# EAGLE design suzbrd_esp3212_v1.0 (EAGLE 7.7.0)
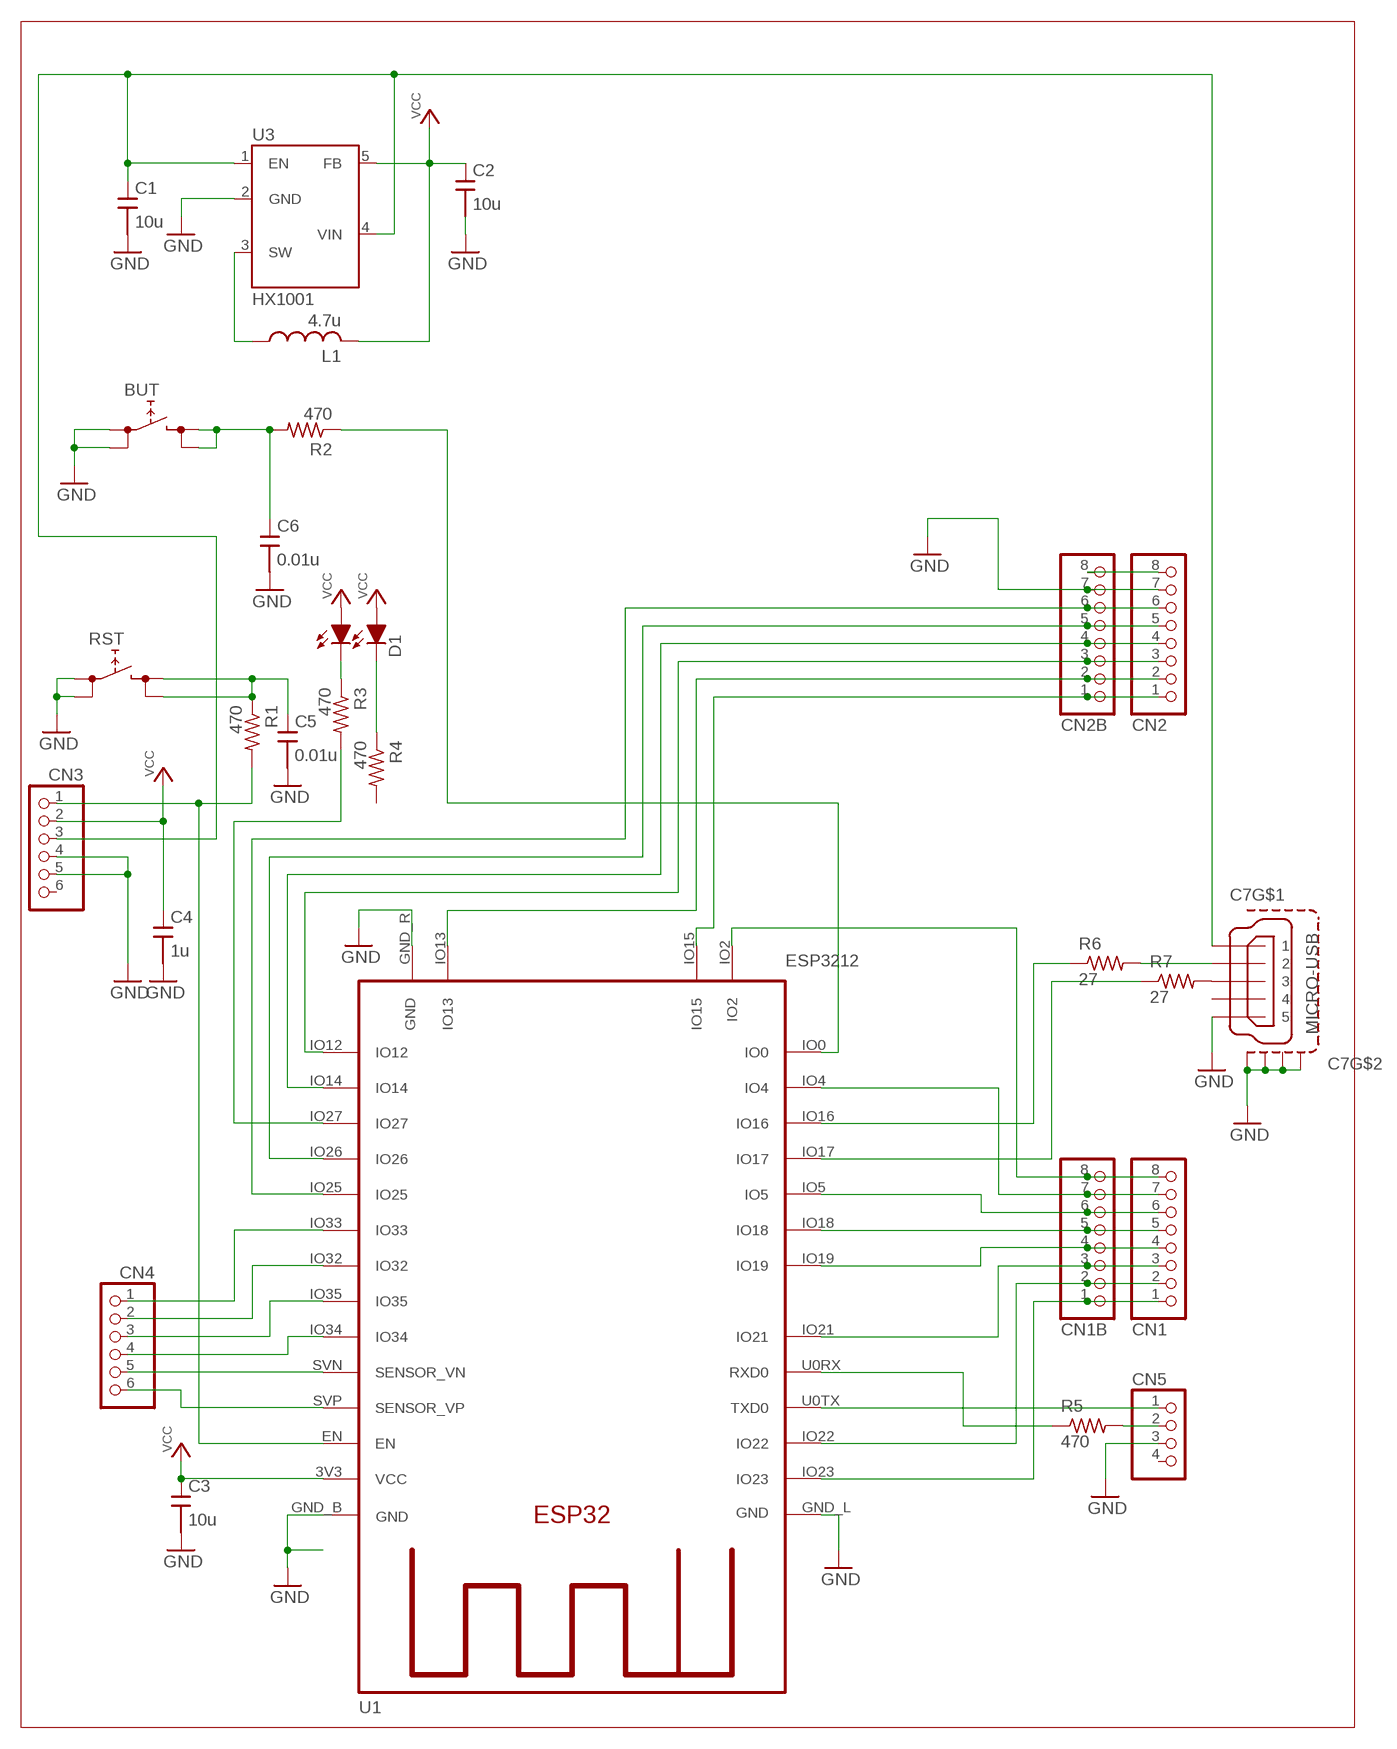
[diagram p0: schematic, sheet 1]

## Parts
BUT  TACTSWSMD+  [TACTSW/SMD+]
C1  10u  C/SMDC2012  [C2012]
C2  10u  C/SMDC2012  [C2012]
C3  10u  C/SMDC2012  [C2012]
C4  1u  C/SMDC2012  [C2012]
C5  0.01u  C/SMDC2012  [C2012]
C6  0.01u  C/SMDC2012  [C2012]
C7  MICRO-USB  [ZX62R]
CN1  PINHDR8  [PINHDR1X8]
CN1B  PINHDR81.0  [PINHDR1X8_1.0]
CN2  PINHDR8  [PINHDR1X8]
CN2B  PINHDR81.0  [PINHDR1X8_1.0]
CN3  PINHDR61.0  [PINHDR1X6_1.0]
CN4  PINHDR61.0  [PINHDR1X6_1.0]
CN5  CONN4N  [PINHDR1X4]
D1  SEC2XX4  [LED3025]
L1  4.7u  L/SMDNRG4026  [NRG4026]
R1  470  R/SMDR2012  [R2012]
R2  470  R/SMDR2012  [R2012]
R3  470  R/SMDR2012  [R2012]
R4  470  R/SMDR2012  [R2012]
R5  470  R/SMDR2012  [R2012]
R6  27  R/SMDR2012  [R2012]
R7  27  R/SMDR2012  [R2012]
RST  TACTSWSMD+  [TACTSW/SMD+]
U1  ESP3212  [ESP3212]
U3  HX1001  [SOT235]

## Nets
5V: C1.1 C7.1 CN3.3 U3.1(EN) U3.4(VIN)
EN: CN3.1 R1.2 U1.EN
GND: BUT.1 BUT.2 C1.2 C2.2 C3.2 C4.2 C5.2 C6.2 C7.5 C7.M1(S1) C7.M2(S2) C7.M3(S3) C7.M4(S4) CN2.7 CN2B.7 CN3.4 CN3.5 CN5.3 RST.1 RST.2 U1.GND_B(GND) U1.GND_L(GND) U1.GND_R(GND) U3.2(GND)
IO0: R2.1 U1.IO0
IO2: CN1.8 CN1B.8 U1.IO2
IO4: CN1.7 CN1B.7 U1.IO4
IO5: CN1.6 CN1B.6 U1.IO5
IO12: CN2.3 CN2B.3 U1.IO12
IO13: CN2.2 CN2B.2 U1.IO13
IO14: CN2.4 CN2B.4 U1.IO14
IO15: CN2.1 CN2B.1 U1.IO15
IO16: R6.1 U1.IO16
IO17: R7.1 U1.IO17
IO18: CN1.5 CN1B.5 U1.IO18
IO19: CN1.4 CN1B.4 U1.IO19
IO21: CN1.3 CN1B.3 U1.IO21
IO22: CN1.2 CN1B.2 U1.IO22
IO23: CN1.1 CN1B.1 U1.IO23
IO25: CN2.6 CN2B.6 U1.IO25
IO26: CN2.5 CN2B.5 U1.IO26
IO27: R3.2 U1.IO27
IO32: CN4.2 U1.IO32
IO33: CN4.1 U1.IO33
IO34: CN4.4 U1.IO34
IO35: CN4.3 U1.IO35
N$1: C7.3 R7.2
N$3: CN5.2 R5.2
N$21: C5.1 R1.1 RST.3 RST.4
N$25: D1.2(C1) R3.1
N$26: D1.1(C0) R4.1
N$32: C7.2 R6.2
N$36: CN2.8 CN2B.8
N$37: BUT.3 BUT.4 C6.1 R2.2
RXD0: R5.1 U1.U0RX(RXD0)
SW: L1.1 U3.3(SW)
TXD0: CN5.1 U1.U0TX(TXD0)
VCC: C2.1 C3.1 C4.1 CN3.2 D1.3(A1) D1.4(A0) L1.2 U1.3V3(VCC) U3.5(FB)
VN: CN4.5 U1.SVN(SENSOR_VN)
VP: CN4.6 U1.SVP(SENSOR_VP)
Unconnected: C7.4 CN3.6 CN5.4 R4.2

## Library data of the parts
BUT RST = SRT162-010:TACTSW: 4pin tactsw (1,2 - 3,4)
C1-C6 = SRT162-010:C/SMD
C7 = SRT162-020:MICRO-USB
CN1 CN1B CN2 CN2B = SRT162-010:PINHDR8
CN3 CN4 = SRT162-010:PINHDR6
CN5 = SRT162-010:CONN4: connector 4
D1 = SRT162-010:SEC2XX4
L1 = SRT162-010:L/SMD: VLF4012AT
R1-R7 = SRT162-010:R/SMD
U1 = SRT162-020:ESP3212
U3 = SRT162-010:HX1001

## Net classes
1 Power: width 0.381 mm, clearance 0.203 mm to class 0

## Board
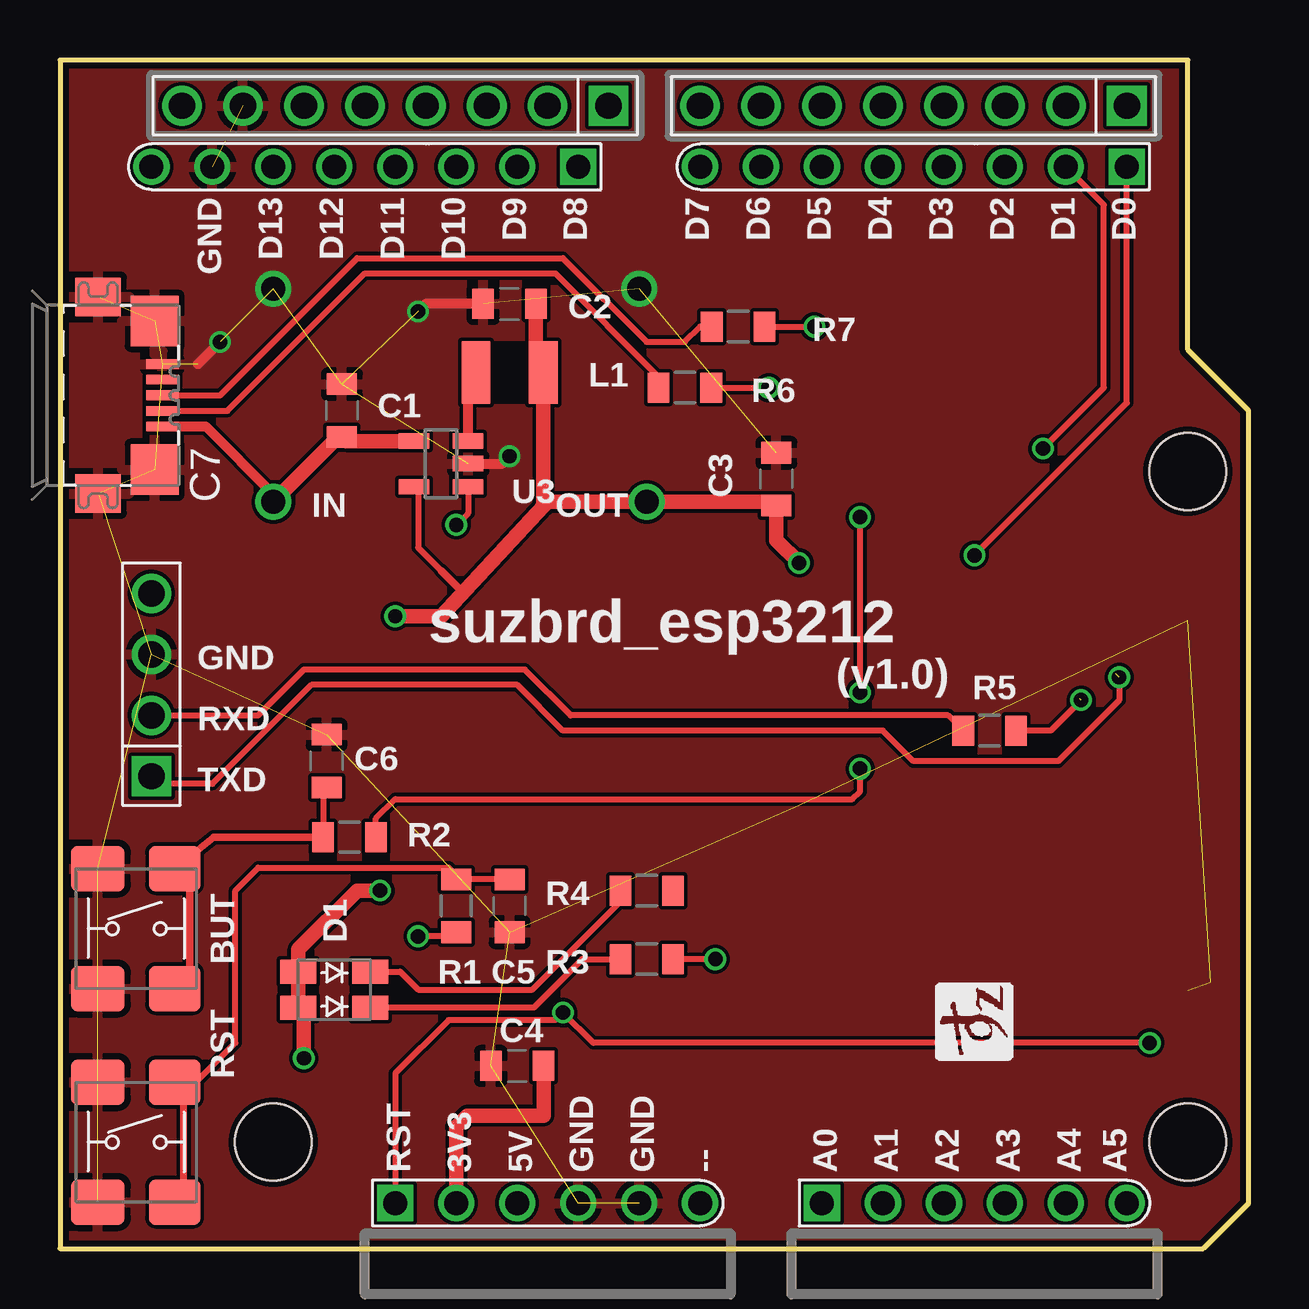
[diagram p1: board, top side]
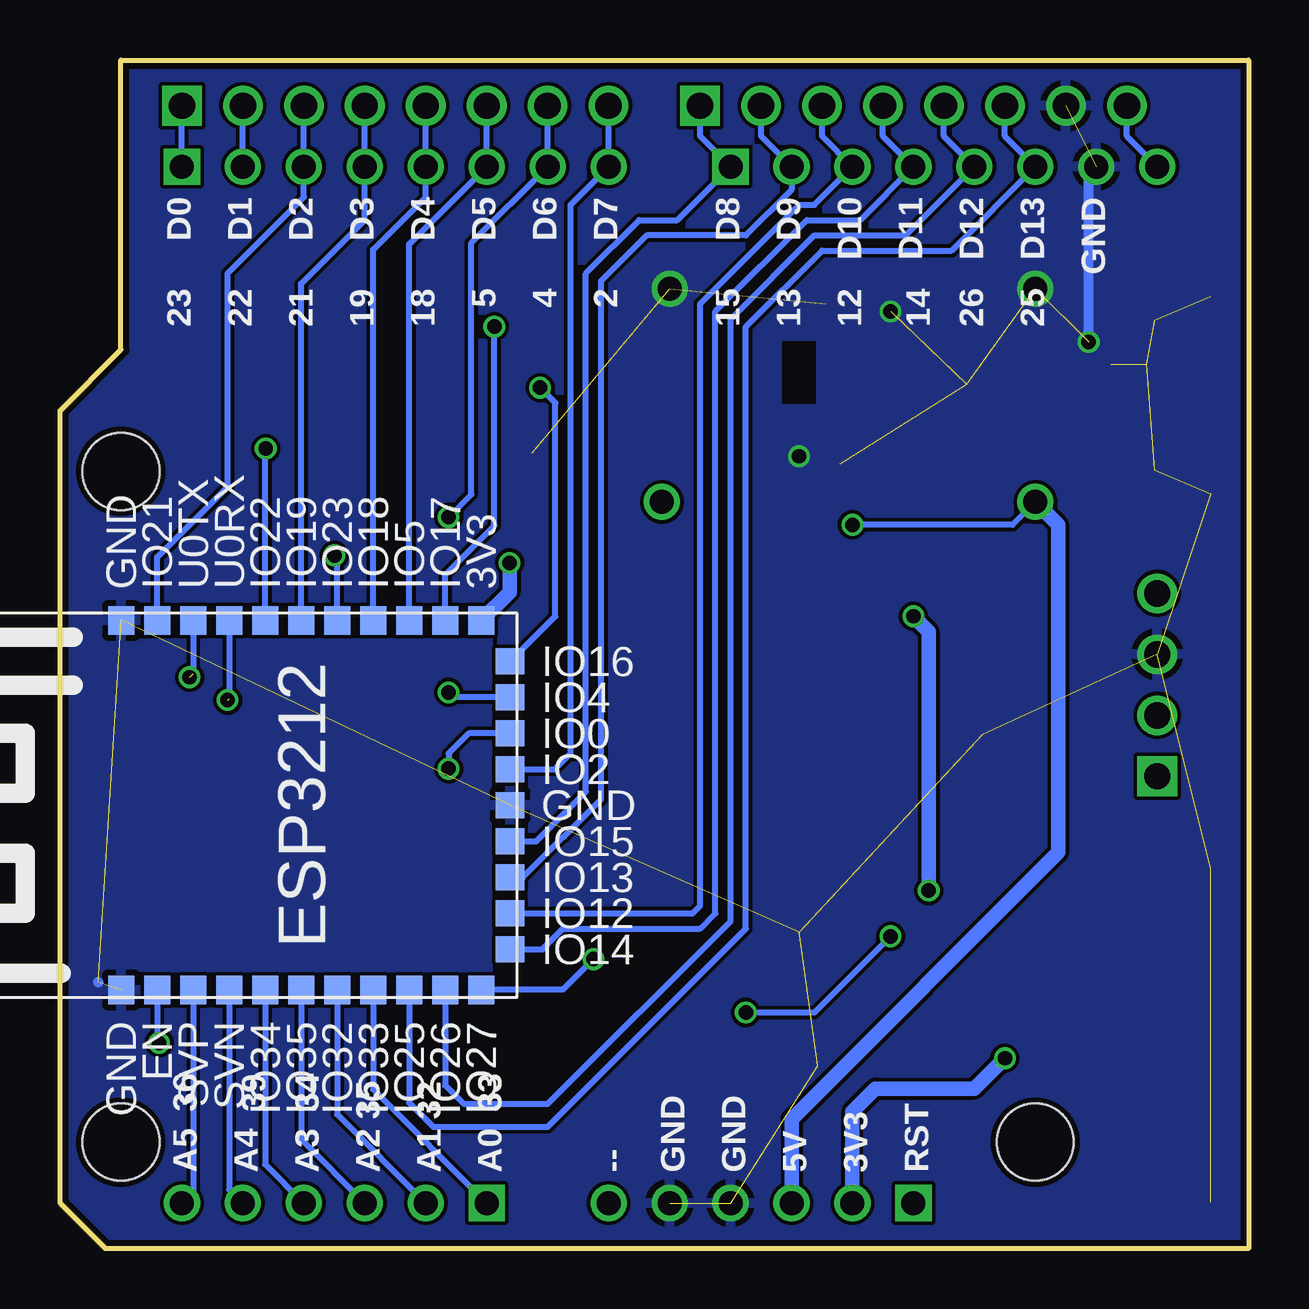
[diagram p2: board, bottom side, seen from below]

Size 49.53 x 49.53 mm. Coordinates in mm from the lower left corner, seen from the top.
Outline: 0,0 47.62,0 49.53,1.91 49.53,34.93 46.99,37.47 46.99,49.53 0,49.53 0,0
Copper layers (1*16): Top 0.035mm / dielectric 1.5mm / Bottom 0.035mm
Design rules "SeeedStudio": minimum track width 6mil, minimum drill 12mil, track to track 6mil, track to pad 6mil, pad to pad 6mil, via to via 6mil, smd to smd 0mil, copper to edge 10mil, drill to drill 10mil, minimum pad ring 10mil, minimum via ring 6mil, stop-mask expansion 2mil, vias tented up to drill 25mil, thermal gap 10mil
Holes 3.2 mm at 46.99,4.45 46.99,32.39 8.89,4.45
vRestrict: area 1.9,41.9 to 45.7,44.5; area 12.7,3.2 to 44.4,5.1

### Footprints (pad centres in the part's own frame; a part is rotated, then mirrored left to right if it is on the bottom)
TACTSW/SMD+ = smd 2.25 x 1.9: 1 -1.6,2.5; 2 -1.6,-2.5 | smd 2.15 x 1.9: 3 1.6,2.5; 4 1.6,-2.5
C2012 = smd 0.9 x 1.25: 1 -1.1,0; 2 1.1,0
ZX62R = smd 1.35 x 0.4: 1 2.675,-1.3; 2 2.675,-0.65; 3 2.675,0; 4 2.675,0.65; 5 2.675,1.3 | smd 1.9 x 1.6: M1 0,-4.1; M2 0,4.1 | smd 2 x 2.1: M3 2.35,3.1; M4 2.35,-3.1
PINHDR1X8 = drill 1.1 square: 1 -8.89,0 | drill 1.1: 2 -6.35,0; 3 -3.81,0; 4 -1.27,0; 5 1.27,0; 6 3.81,0; 7 6.35,0; 8 8.89,0
PINHDR1X8_1.0 = drill 1 square: 1 -8.89,0 | drill 1: 2 -6.35,0; 3 -3.81,0; 4 -1.27,0; 5 1.27,0; 6 3.81,0; 7 6.35,0; 8 8.89,0
PINHDR1X6_1.0 = drill 1 square: 1 -6.35,0 | drill 1: 2 -3.81,0; 3 -1.27,0; 4 1.27,0; 5 3.81,0; 6 6.35,0
PINHDR1X4 = drill 1.1 square: 1 -3.81,0 | drill 1.1: 2 -1.27,0; 3 1.27,0; 4 3.81,0
LED3025 = smd 1.5 x 1: 1 1.5,0.75; 2 1.5,-0.75; 3 -1.5,-0.75; 4 -1.5,0.75
NRG4026 = smd 1.2 x 2.6: 1 -1.4,0; 2 1.4,0
R2012 = smd 0.9 x 1.25: 1 -1.1,0; 2 1.1,0
ESP3212 = smd 1.2 x 1.1: 3V3 8.08,-7.39; EN -7.32,6.11; GND_L -7.32,7.61; GND_R 8.08,7.61; IO5 8.08,-4.39; IO17 8.08,-5.89; IO18 8.08,-2.89; IO19 8.08,0.11; IO21 8.08,6.11; IO22 8.08,1.61; IO23 8.08,-1.39; IO25 -7.32,-4.39; IO26 -7.32,-5.89; IO27 -7.32,-7.39; IO32 -7.32,-1.39; IO33 -7.32,-2.89; IO34 -7.32,1.61; IO35 -7.32,0.11; SVN -7.32,3.11; SVP -7.32,4.61; U0RX 8.08,3.11; U0TX 8.08,4.61 | smd 1.1 x 1.2: GND_B 0.38,-8.59; IO0 3.38,-8.59; IO2 1.88,-8.59; IO4 4.88,-8.59; IO12 -4.12,-8.59; IO13 -2.62,-8.59; IO14 -5.62,-8.59; IO15 -1.12,-8.59; IO16 6.38,-8.59
SOT235 = smd 0.635 x 1.27: 1 -0.95,-1.125; 2 0.013,-1.135; 3 0.95,-1.125; 4 0.95,1.125; 5 -0.95,1.125

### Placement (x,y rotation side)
BUT  3.18,13.34 0 top
C1  11.75,34.93 90 top
C2  18.73,39.37 180 top
C3  29.84,32.07 90 top
C4  19.05,7.62 180 top
C5  18.73,14.29 270 top
C6  11.11,20.32 90 top
C7  1.59,35.56 0 top
CN1  35.56,47.62 180 top
CN1B  35.56,45.09 180 top
CN2  13.97,47.62 180 top
CN2B  12.7,45.09 180 top
CN3  20.32,1.91 0 top
CN4  38.1,1.91 0 top
CN5  3.81,23.5 90 top
D1  11.43,10.8 0 top
L1  18.73,36.51 0 top
R1  16.51,14.29 270 top
R2  12.07,17.14 180 top
R3  24.45,12.07 0 top
R4  24.45,14.92 0 top
R5  38.73,21.59 180 top
R6  26.04,35.88 180 top
R7  28.26,38.42 180 top
RST  3.18,4.45 0 top
U1  39.37,18.1 90 bottom
U3  15.88,32.7 90 top

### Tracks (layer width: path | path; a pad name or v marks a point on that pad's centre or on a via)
5V  (via drill 0.6, 1)
  Top 0.254: U3.1 17,30.65 v16.51,30.16
  Top 0.406: v8.89,31.11 8.89,31.43 6.06,34.26 C7.1
  Top 0.61: v8.89,31.11 11.6,33.83 C1.1 11.92,33.65 U3.4
  Bottom 0.254: v8.89,31.11 9.84,30.16 v16.51,30.16
  Bottom 0.61: CN3.3 19.05,5.4 7.94,16.51 7.94,30.16 v8.89,31.11
EN  (via drill 0.6)
  Top 0.254: 13.93,1.95 CN3.1 13.97,7.3 16.19,9.52 20.64,9.52 v20.96,9.84 22.23,8.57 v45.4,8.57 | R1.2 16.34,13.02 v14.92,13.02
  Bottom 0.254: v14.92,13.02 18.1,9.84 v20.96,9.84 | U1.EN 45.48,8.65 v45.4,8.57
  Bottom 0.3: CN3.1
GND  (via drill 0.6, 1)  (26 unrouted)
  Top 0.406: 5.74,36.86 v6.67,37.78 | U3.2 18.43,32.72 v18.73,33.02 | C2.2 15.24,39.37 v14.92,39.05
  Bottom 0.406: 47.93,11.1 47.94,11.11 | v6.67,37.78 6.67,44.77 CN2B.7
  other vias: 8.89,40.01 24.13,40.01
  pour Bottom: -0.64,50.17 52.07,50.17 52.07,-3.17 -0.64,-3.17
  pour Top: -1.27,50.8 53.34,50.8 53.34,-3.81 -1.27,-3.81
IO0  (via drill 0.6)
  Top 0.254: R2.1 13.17,17.93 13.97,18.73 33.02,18.73 33.34,19.05 v33.34,20
  Bottom 0.254: U1.IO0 32.5,21.48 33.34,20.64 v33.34,20
IO2
  Bottom 0.254: CN1.8 CN1B.8 28.26,43.5 28.26,20.64 28.92,19.98 U1.IO2
IO4  (via drill 0.6)
  Top 0.254: v33.34,23.18 v33.34,30.48
  Bottom 0.254: CN1.7 CN1B.7 32.38,41.91 32.38,31.43 v33.34,30.48 | U1.IO4 33.14,22.98 v33.34,23.18
IO5
  Bottom 0.254: 31.75,44.77 CN1B.6 | CN1B.6 CN1.6 | U1.IO5 34.98,41.86 CN1B.6
IO12
  Bottom 0.254: CN2.3 17.78,46.36 CN2B.3 18.1,43.5 18.73,43.5 22.86,39.37 22.86,14.29 23.17,13.98 U1.IO12
IO13
  Bottom 0.254: CN2.2 20.32,46.36 CN2B.2 19.05,44.13 20.96,42.23 25.08,42.23 26.99,40.32 26.99,18.73 30.24,15.48 U1.IO13
IO14
  Bottom 0.254: CN2.4 15.24,46.36 CN2B.4 16.19,42.86 18.41,42.86 22.23,39.05 22.23,13.97 22.86,13.34 28.57,13.34 29.43,12.48 U1.IO14
IO15
  Bottom 0.254: CN2.1 22.86,46.36 CN2B.1 23.81,42.86 25.4,42.86 27.62,40.64 27.62,19.05 29.7,16.98 U1.IO15
IO16  (via drill 0.6)
  Top 0.254: R6.1 v29.53,35.88
  Bottom 0.254: U1.IO16 30.77,24.48 28.89,26.35 28.89,35.24 v29.53,35.88
IO17  (via drill 0.6)
  Top 0.254: R7.1 v31.43,38.42
  Bottom 0.254: U1.IO17 33.48,28.08 31.43,30.13 v31.43,38.42
IO18
  Bottom 0.254: CN1.5 CN1B.5 34.29,43.82 36.48,41.62 U1.IO18
IO19
  Bottom 0.254: CN1.4 CN1B.4 36.83,42.86 39.48,40.21 U1.IO19
IO21
  Bottom 0.254: CN1.3 CN1B.3 39.37,43.82 42.54,40.64 42.54,31.75 45.48,28.81 U1.IO21
IO22  (via drill 0.6)
  Top 0.254: v40.96,33.34 43.5,35.88 43.5,43.5 CN1B.2
  Bottom 0.254: CN1B.2 CN1.2 | U1.IO22 40.98,33.32 v40.96,33.34
IO23  (via drill 0.6)
  Top 0.254: v38.1,28.89 44.45,35.24 CN1B.1
  Bottom 0.254: CN1B.1 CN1.1 | U1.IO23 37.98,28.77 v38.1,28.89
IO25
  Bottom 0.254: CN2.6 10.16,46.36 CN2B.6 12.38,41.59 17.78,41.59 20.96,38.42 20.96,13.34 29.21,5.08 33.97,5.08 34.98,6.09 U1.IO25
IO26
  Bottom 0.254: CN2.5 12.7,46.36 CN2B.5 14.29,42.23 18.1,42.23 21.59,38.73 21.59,13.65 29.21,6.03 32.7,6.03 33.48,6.81 U1.IO26
IO27  (via drill 0.6)
  Top 0.254: v27.3,12.07 R3.2
  Bottom 0.254: v27.3,12.07 28.57,10.8 31.96,10.8 U1.IO27
IO32
  Bottom 0.254: U1.IO32 37.98,5.59 CN4.2
IO33
  Bottom 0.254: U1.IO33 36.48,6.64 CN4.1
IO34
  Bottom 0.254: U1.IO34 40.98,3.52 CN4.4
IO35
  Bottom 0.254: U1.IO35 39.48,4.56 CN4.3
N$1
  Top 0.254: C7.3 6.67,35.56 12.38,41.28 20.96,41.28 24.45,37.78 26.04,37.78 26.67,38.42 R7.2
N$3
  Top 0.254: CN5.2 8.26,22.22 10.16,24.13 19.37,24.13 21.27,22.22 37,22.22 R5.2
N$21
  Top 0.254: 5.16,6.27 5.16,6.43 7.3,8.57 7.3,14.92 8.26,15.88 16.19,15.88 16.83,15.24 16.66,15.24 R1.1 C5.1
  Top 0.3: RST.4 5.16,2.14 5.16,6.27 RST.3
N$25
  Top 0.254: D1.2 19.74,10.05 21.76,12.07 R3.1
N$26
  Top 0.254: D1.1 14.17,11.55 14.92,10.8 19.68,10.8 23.35,14.46 R4.1
N$32
  Top 0.254: C7.2 6.97,34.91 12.7,40.64 20.64,40.64 24.93,36.34 R6.2
N$36
  Bottom 0.254: CN2B.8 5.08,46.36 CN2.8
N$37
  Top 0.152: BUT.4 4.84,10.88 5.32,10.88 5.32,11.03 5.4,11.11
  Top 0.254: C6.1 10.96,19.07 R2.2
  Top 0.305: R2.2 6.4,17.14 BUT.3 5.4,15.84 5.4,11.11
RXD0  (via drill 0.6)  (1 unrouted)
  Top 0.254: v42.54,22.86 41.27,21.59 R5.1
  Bottom 0.254: U1.U0RX 42.48,22.93
SW
  Top 0.406: U3.3 17,36.18 L1.1
TXD0  (via drill 0.6)  (1 unrouted)
  Top 0.254: CN5.1 4.13,19.37 6.35,19.37 10.48,23.5 19.05,23.5 20.96,21.59 34.29,21.59 35.56,20.32 41.59,20.32 44.13,22.86 v44.13,23.81
  Bottom 0.254: U1.U0TX 43.98,23.96
VCC  (via drill 0.6, 1)
  Top 0.254: U3.5 14.92,31.58 14.92,29.21 15.88,28.26
  Top 0.305: 15.88,28.26 16.65,27.48 16.93,27.48
  Top 0.406: 10.16,9.82 D1.3 | 19.83,36.81 L1.2 | 14.29,26.35 v13.97,26.35
  Top 0.61: C4.1 20.15,5.55 16.98,5.55 16.51,5.08 CN3.2 | v10.16,7.94 10.16,9.82 | D1.3 D1.4 9.93,12.47 12.38,14.92 v13.34,14.92 | C2.1 19.83,36.81 | L1.2 20.13,30.93 | 20.13,30.93 16.93,27.48 15.88,26.35 14.29,26.35 | 20.13,30.93 20.32,31.11 v24.45,31.11 29.7,31.11 C3.1 29.84,29.53 v30.8,28.57
  Bottom 0.61: CN3.2 16.51,5.72 15.56,6.67 11.43,6.67 v10.16,7.94 | v13.97,26.35 13.34,25.72 v13.34,14.92 | v30.8,28.57 30.8,27.36 U1.3V3
VN
  Bottom 0.254: U1.SVN 42.48,2.48 CN4.5
VP
  Bottom 0.254: 44.12,2.24 CN4.6 43.98,2.38 U1.SVP

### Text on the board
tPlace: GND | D13 | D12 | D11 | D10 | D9 | D8 | D7 | D6 | D5 | D4 | D3 | D2 | D1 | D0 | IN | OUT | suzbrd_esp3212 | (v1.0) | GND | RXD | TXD | RST | 3V3 | 5V | GND | GND | -- | A0 | A1 | A2 | A3 | A4 | A5
bPlace: GND | D13 | D12 | D11 | D10 | D9 | D8 | D7 | D6 | D5 | D4 | D3 | D2 | D1 | D0 | 25 | 26 | 14 | 12 | 13 | 15 | 2 | 4 | 5 | 18 | 19 | 21 | 22 | 23 | 33 | 32 | 35 | 34 | 39 | 36 | RST | 3V3 | 5V | GND | GND | -- | A0 | A1 | A2 | A3 | A4 | A5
